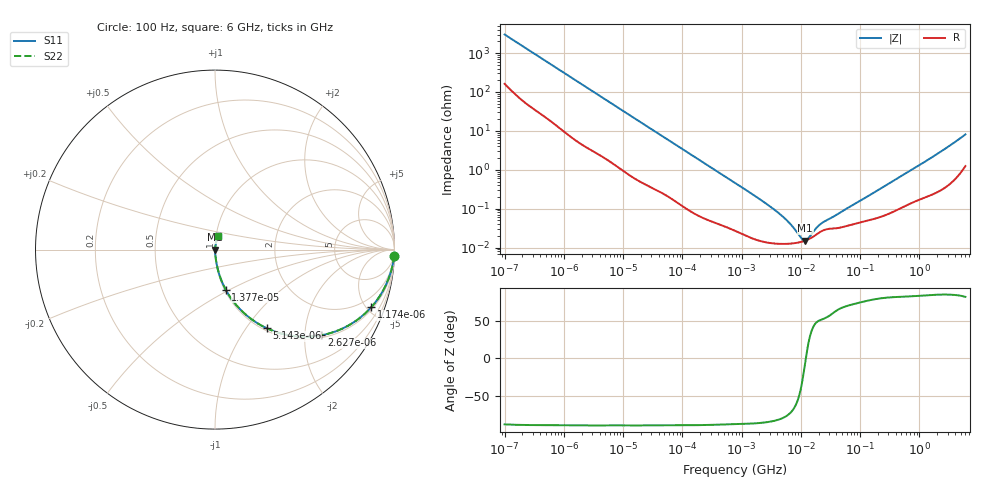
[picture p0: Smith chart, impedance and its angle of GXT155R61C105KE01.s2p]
!Murata Part Number: GXT155R61C105KE01
!These Parameters are Measured in Series Mode Connection
!Data Generated on Jan 08, 2026
!  o--ll--o
!Port1  Port2
!  o------o
!Operation Temp=25[degC], DC Bias Voltage=0[V]
!Freq. Start=100[Hz] Stop=6[GHz] 401[Steps]
# Hz S RI R 50
!Freq.(Hz) S11(Real) S11(Imag) S21(Real) S21(Imag) S12(Real) S12(Imag) S22(Real) S22(Imag)
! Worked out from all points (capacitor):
!   401 points, 100 Hz to 6 GHz, reference 50 ohm
!   read as one part in series: C = 526 nF near 109 Hz
!   lowest |Z| = 15.2 mohm at 11.89 MHz (marker M1)
!   series resonance near 12.15 MHz, so ESL is about 330 pH
!   S11 on the Smith chart (normalised r, x): 100 Hz: 4, -60; 1.174 kHz: 1.16, -5.37; 2.627 kHz: 1.07, -2.43; 5.143 kHz: 1.04, -1.26; 13.77 kHz: 1.01, -0.48; 6 GHz: 1.02, +0.16
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100  0.9971 -0.033  0.00288 0.033  0.00288 0.033  0.9971 -0.033
401  0.979 -0.1266  0.021 0.1266  0.021 0.1266  0.979 -0.1266
1174  0.8711 -0.3206  0.1289 0.3206  0.1289 0.3206  0.8711 -0.3206
2008  0.7091 -0.4403  0.2909 0.4403  0.2909 0.4403  0.7091 -0.4403
2627  0.5931 -0.4772  0.4069 0.4772  0.4069 0.4772  0.5931 -0.4772
5143  0.2888 -0.4384  0.7112 0.4384  0.7112 0.4384  0.2888 -0.4384
8047  0.1482 -0.341  0.8518 0.341  0.8518 0.341  0.1482 -0.341
13772  0.0596 -0.223  0.9404 0.223  0.9404 0.223  0.0596 -0.223
40335  0.00958 -0.082  0.9904 0.082  0.9904 0.082  0.00958 -0.082
129199  0.00161 -0.0265  0.9984 0.0265  0.9984 0.0265  0.00161 -0.0265
774597  0.000291 -0.00459  0.9997 0.00459  0.9997 0.00459  0.000291 -0.00459
4246196  0.000126 -0.000758  0.9999 0.000758  0.9999 0.000758  0.000126 -0.000758
6644369  0.000127 -0.000386  0.9999 0.000386  0.9999 0.000386  0.000127 -0.000386
1.039699e7  0.000142 -9.37e-05  0.9999 9.37e-05  0.9999 9.37e-05  0.000142 -9.37e-05
1.189169e7  0.000151 -1.28e-05  0.9998 1.28e-05  0.9998 1.28e-05  0.000151 -1.28e-05
1.300572e7  0.00016 4.04e-05  0.9998 -4.04e-05  0.9998 -4.04e-05  0.00016 4.04e-05
1.555665e7  0.000184 0.000145  0.9998 -0.000145  0.9998 -0.000145  0.000184 0.000145
1.946e7  0.000231 0.000267  0.9998 -0.000267  0.9998 -0.000267  0.000231 0.000267
2.327686e7  0.000272 0.000345  0.9997 -0.000345  0.9997 -0.000345  0.000272 0.000345
3.124326e8  0.00077 0.00445  0.9992 -0.00445  0.9992 -0.00445  0.00077 0.00445
1.637704e9  0.00272 0.0208  0.9973 -0.0208  0.9973 -0.0208  0.00272 0.0208
6e9  0.0185 0.078  0.9815 -0.078  0.9815 -0.078  0.0185 0.078
